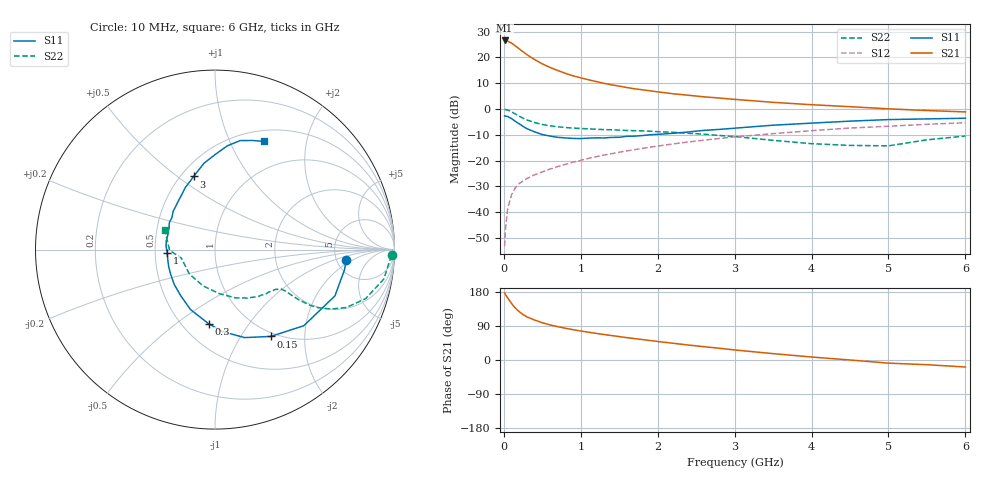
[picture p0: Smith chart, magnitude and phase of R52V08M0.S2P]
! SIEMENS Small Signal Semiconductors
! BFR183
! Si NPN RF Bipolar Junction Transistor in SOT23
! VCE = 2 V  IC = 8 mA
! Common Emitter S-Parameters:  May  1996
# GHz  S  MA  R  50
!  f  S11  S21  S12  S22
! GHz  MAG  ANG  MAG  ANG  MAG  ANG  MAG  ANG
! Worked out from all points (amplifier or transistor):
!   36 points, 10 MHz to 6 GHz, reference 50 ohm
!   highest |S21| = 26.6 dB at 10 MHz (marker M1)
!   |S21| within 3 dB of that: start of sweep to 188.7 MHz
!   unconditionally stable (mu >= 1): 815.1 MHz to 2.534 GHz
!   at 250 MHz: K = 0.56, MSG = 25.0 dB, |S12| = -27.9 dB
!   at 1.4 GHz: K = 1.06, MAG = 11.8 dB, |S12| = -17.3 dB
!   at 6 GHz: K = 0.90, MSG = 2.1 dB, |S12| = -5.3 dB
!   lowest NFmin = 1.30 dB at 450 MHz
!   S11 on the Smith chart (normalised r, x): 10 MHz: 6.15, -1.51; 150 MHz: 0.94, -1.36; 300 MHz: 0.67, -0.67; 1 GHz: 0.58, -0.02; 3 GHz: 0.58, +0.57; 6 GHz: 0.63, +1.35
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0.01  0.7344 -4.4  21.28 176.8  0.0022 87.3  0.9854 -1.9
0.02  0.7302 -8.9  21.1 173.1  0.0046 89.5  0.9739 -4.0
0.05  0.7163 -21.1  20.6 163.7  0.0118 80.8  0.9548 -9.9
0.1  0.6517 -40.6  18.95 149.2  0.0219 72.7  0.8829 -18.0
0.15  0.5748 -57.3  16.65 136.7  0.0298 65.9  0.7998 -23.8
0.2  0.5173 -71.4  14.63 127.5  0.0361 62.7  0.7269 -27.1
0.25  0.4598 -84.4  12.82 119.7  0.0403 60.7  0.6624 -29.3
0.3  0.4151 -94.8  11.31 113.9  0.045 60.0  0.6125 -30.4
0.4  0.3609 -112.2  9.071 105.5  0.0531 60.1  0.546 -30.9
0.5  0.3198 -126.8  7.481 98.2  0.0605 60.4  0.5013 -30.8
0.6  0.2987 -139.5  6.393 92.7  0.0685 61.4  0.4716 -30.6
0.7  0.2828 -150.9  5.573 88.0  0.0767 62.4  0.4526 -30.5
0.8  0.2752 -159.4  4.906 83.8  0.0847 62.3  0.4374 -30.7
1  0.2671 -176.3  4.01 76.6  0.1011 62.8  0.4197 -31.4
1.1  0.2731 176.6  3.685 73.4  0.1102 63.0  0.412 -32.5
1.6  0.2957 149.3  2.604 58.9  0.1544 61.3  0.3832 -37.9
2.2  0.3385 127.3  1.973 44.2  0.2105 57.1  0.3538 -47.9
3  0.4247 106.3  1.536 26.5  0.288 49.0  0.2929 -66.8
3.5  0.4855 97.2  1.346 16.8  0.3332 42.9  0.2471 -84.1
4.5  0.5818 83.3  1.109 0.0  0.4276 30.4  0.197 -136.5
5.5  0.6433 70.9  0.933 -12.4  0.5054 18.3  0.253 -179.2
6  0.662 65.5  0.878 -18.5  0.5416 10.4  0.2994 158.9
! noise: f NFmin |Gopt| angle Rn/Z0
0.45  1.3  0.17  43  0.21
0.9  1.35  0.21  115  0.2
1.8  2.05  0.33  -177  0.14
